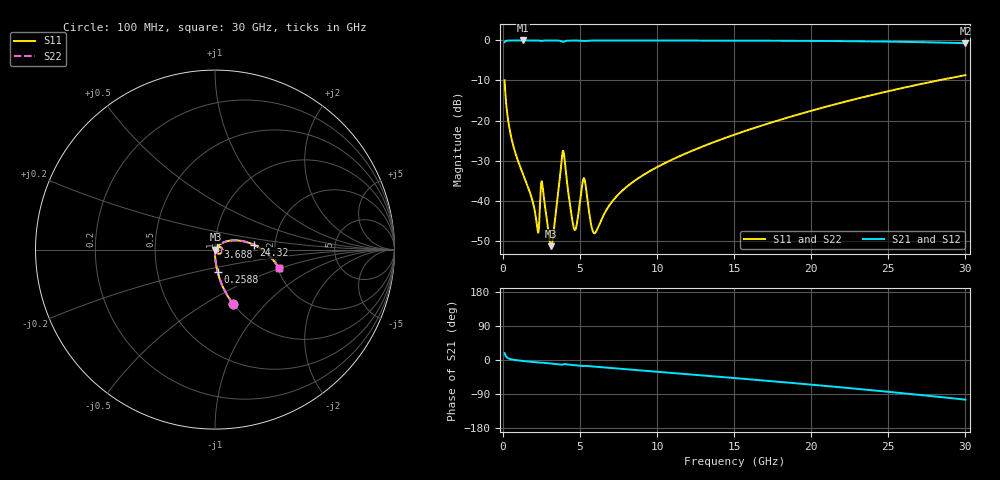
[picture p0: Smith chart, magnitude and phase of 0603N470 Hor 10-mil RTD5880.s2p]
# GHz S MA R 50
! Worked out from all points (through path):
!   3201 points, 100 MHz to 30 GHz, reference 50 ohm
!   highest |S21| = -0.01 dB at 1.315 GHz (marker M1); lowest = -0.7 dB at 30 GHz (marker M2)
!   group delay of S21, straight-line fit = 9.7 ps
!   lowest |S11| = -51.4 dB at 3.118 GHz (marker M3), VSWR 1.01, Z = 50.3 - j0.067 ohm
!   |S11| at or under -10 dB: 100.5 MHz to 28.22 GHz (28.12 GHz wide, 199 % of centre)
!   |S22| runs from -51.4 to -8.7 dB; largest |S21 - S12| = 0
!   S11 on the Smith chart (normalised r, x): 100 MHz: 1.00, -0.67; 258.8 MHz: 1.00, -0.26; 3.688 GHz: 1.03, +0.03; 24.32 GHz: 1.54, +0.09; 30 GHz: 2.03, -0.47
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0.1  0.3177 -71.7  0.9478 18.2  0.9478 18.2  0.3177 -71.7
0.2588437  0.1277 -83.2  0.9913 6.6  0.9913 6.6  0.1277 -83.2
0.62325  0.05171 -88.1  0.9979 1.1  0.9979 1.1  0.05171 -88.1
1.314688  0.02097 -89.7  0.9987 -2.7  0.9987 -2.7  0.02097 -89.7
2.211688  0.004669 -63.6  0.9974 -6.4  0.9974 -6.4  0.004669 -63.6
2.576094  0.01431 -59.3  0.9911 -7.0  0.9911 -7.0  0.01431 -59.3
3.118031  0.0027 -14.3  0.9973 -9.3  0.9973 -9.3  0.0027 -14.3
3.276875  0.004005 31.1  0.9969 -9.9  0.9969 -9.9  0.004005 31.1
3.688  0.01934 44.6  0.9892 -11.9  0.9892 -11.9  0.01934 44.6
3.949625  0.03827 -31.7  0.964 -11.0  0.964 -11.0  0.03827 -31.7
4.641063  0.004319 -21.0  0.9956 -13.8  0.9956 -13.8  0.004319 -21.0
5.089563  0.01356 22.0  0.9892 -15.6  0.9892 -15.6  0.01356 22.0
5.304469  0.01786 -25.3  0.9823 -15.6  0.9823 -15.6  0.01786 -25.3
5.715594  0.004994 -34.0  0.9951 -16.9  0.9951 -16.9  0.004994 -34.0
5.958531  0.003934 2.7  0.9962 -17.8  0.9962 -17.8  0.003934 2.7
7.472219  0.01189 53.0  0.9969 -22.8  0.9969 -22.8  0.01189 53.0
10.06978  0.02667 51.9  0.9963 -31.3  0.9963 -31.3  0.02667 51.9
15.05  0.06695 38.9  0.9936 -47.7  0.9936 -47.7  0.06695 38.9
20.03956  0.133 22.7  0.9859 -65.2  0.9859 -65.2  0.133 22.7
24.319  0.2165 7.2  0.9701 -81.3  0.9701 -81.3  0.2165 7.2
25.01978  0.2328 4.5  0.9662 -84.0  0.9662 -84.0  0.2328 4.5
30  0.3684 -15.7  0.9221 -104.6  0.9221 -104.6  0.3684 -15.7
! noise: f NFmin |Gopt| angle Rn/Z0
0.1  0.000296  0.9195  0.3666  0.0008123
3.417  0.005286  0.8516  10.19  0.007535
6.743  0.006604  0.7765  20.02  0.005864
10.06  0.00833  0.7432  29.64  0.006094
13.39  0.01032  0.7299  39.07  0.006781
16.7  0.01234  0.7234  48.22  0.007415
20.03  0.01443  0.7215  57.09  0.007984
23.35  0.01661  0.7229  65.64  0.00849
26.67  0.01896  0.727  73.9  0.008943
30  0.0215  0.7333  81.85  0.009348
